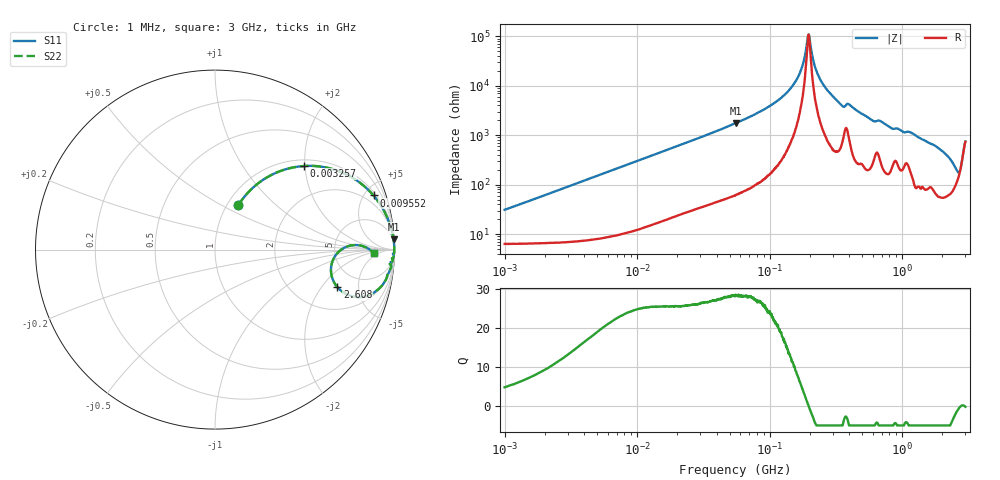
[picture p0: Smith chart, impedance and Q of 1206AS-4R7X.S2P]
!s-Parameter Generated by FASTRON Sdn. Bhd.
!FASTRON P/N : 1206AS-4R7X
!Keysight Technologies: E4991B_MY54100416_A.01.15
!Date created: Thu Nov 16 14:07:03 2023
!Version  : Rev00 Thu Nov 16 14:07:03 2023
!Data & Calibration Information:
!Freq	S11	S21	S12	S22
!PortZ  Port1:50+j0  Port2:50+j0
!When reading reference impedance value at option line is always used.
! Remarks : This data is being provided solely for informational purposes.
# Hz S dB R 50
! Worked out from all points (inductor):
!   1601 points, 1 MHz to 3 GHz, reference 50 ohm
!   read as one part in series: L = 4.84 uH near 1.041 MHz
!   highest Q = 28.3 at 55.32 MHz (marker M1), where L = 5.01 uH
!   self-resonance near 196.2 MHz
!   S11 on the Smith chart (normalised r, x): 1 MHz: 1.13, +0.61; 3.257 MHz: 1.14, +1.97; 9.552 MHz: 1.23, +5.77; 2.608 GHz: 3.39, -2.89; 3 GHz: 16, -3
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1000000  -11.03 62.2  -0.88 -16.0  -0.88 -16.0  -11.03 62.2
3257432  -3.35 43.2  -3.26 -42.7  -3.26 -42.7  -3.35 43.2
3804036  -2.69 39.3  -3.94 -47.1  -3.94 -47.1  -2.69 39.3
9552423  -0.60 18.9  -9.80 -68.8  -9.80 -68.8  -0.60 18.9
1.447069e7  -0.30 12.8  -13.08 -74.9  -13.08 -74.9  -0.30 12.8
5.477226e7  -0.03 3.3  -24.76 -84.7  -24.76 -84.7  -0.03 3.3
5.532317e7  -0.03 3.3  -24.86 -84.7  -24.86 -84.7  -0.03 3.3
1.288778e8  -0.01 0.9  -36.22 -85.6  -36.22 -85.6  -0.01 0.9
1.6718e8  -0.01 0.3  -44.58 -80.8  -44.58 -80.8  -0.01 0.3
1.952332e8  -0.01 0.0  -60.41 -17.9  -60.41 -17.9  -0.01 0.0
2.011837e8  -0.01 -0.0  -58.22 40.8  -58.22 40.8  -0.01 -0.0
2.083556e8  -0.01 -0.1  -52.89 65.6  -52.89 65.6  -0.01 -0.1
2.223601e8  -0.01 -0.3  -46.90 77.6  -46.90 77.6  -0.01 -0.3
2.433181e8  -0.01 -0.4  -42.10 82.0  -42.10 82.0  -0.01 -0.4
3.436571e8  -0.03 -1.4  -32.47 81.0  -32.47 81.0  -0.03 -1.4
3.973271e8  -0.04 -1.3  -32.53 77.3  -32.53 77.3  -0.04 -1.3
7.925923e8  -0.08 -3.8  -23.60 79.9  -23.60 79.9  -0.08 -3.8
1.159346e9  -0.15 -4.9  -21.26 76.3  -21.26 76.3  -0.15 -4.9
2.000286e9  -0.37 -11.4  -14.03 72.2  -14.03 72.2  -0.37 -11.4
2.607784e9  -2.93 -17.1  -8.39 33.4  -8.39 33.4  -2.93 -17.1
2.75535e9  -3.40 -2.3  -9.74 4.8  -9.74 4.8  -3.40 -2.3
3e9  -1.07 -1.4  -18.55 10.2  -18.55 10.2  -1.07 -1.4
